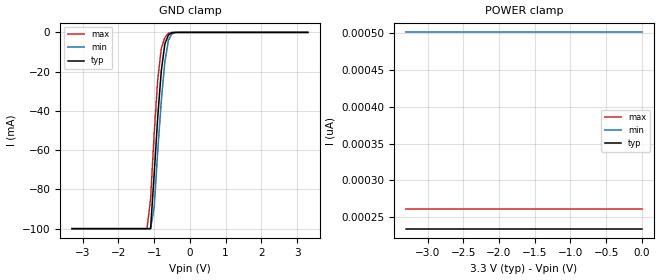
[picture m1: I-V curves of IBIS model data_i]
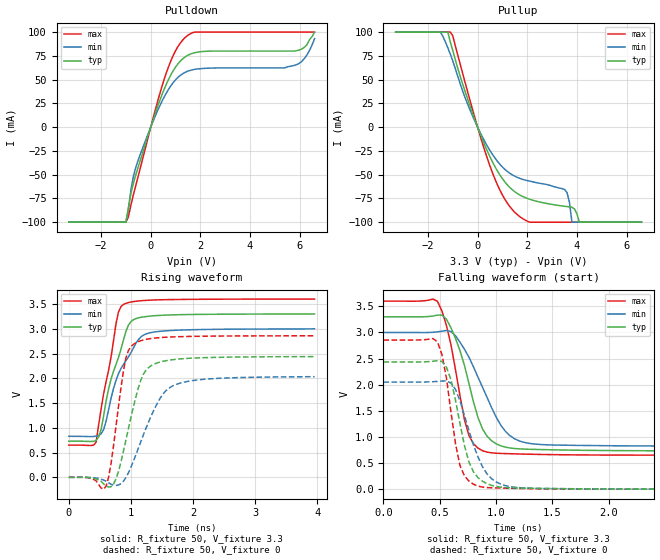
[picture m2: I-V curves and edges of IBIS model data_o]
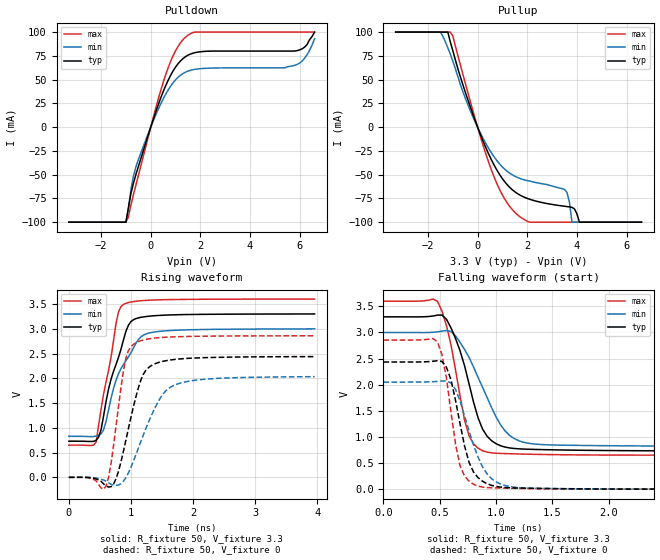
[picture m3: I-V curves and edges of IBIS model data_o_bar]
|   ON Semiconductor Corporation
|   IBIS Model of NL17SZ74DF
|   Single D type Flip-Flop
|   US8 (US) Package Type
[IBIS Ver]   3.2
[Comment Char]   |_char
[File name]   nl17sz74df_c300.ibs
[File Rev]   1.0
[Date]   06/15/04
[Source]
From lab measurements at ON Semiconductor
[Notes]
Created by Duane Mattheisen
Modeling Support Engineer
| This model represents the NL27WZ08DF where 3.0 <= Vcc =< 3.6
[Disclaimer]
ON Semiconductor Corporation hereby grants
the user of this IBIS model a license to use this IBIS
model under the following terms. This license in non-exclusive
and non-transferable. Before using this IBIS model. After reading
the terms and conditions of this license, the user either must accept
these terms, or the IBIS model should be returned to ON within 30 days.
   The user is hereby granted a license to use the
IBIS model. This shall not be construed as a right to sell, or otherwise
profit either by leasing or renting this software.
   The user may modify the IBIS model to suit his specific applications
but rights to derivative works and such modifications shall belong to
ON Semiconductor.
   This IBIS model is provided on an "as is" basis. ON Semiconductor
makes absolutely no warranty with respect to the information contained
herein. By use of this IBIS model, the user assumes full risk as to the
quality and suitability of the model to his particular use, and by using
this model assumes the entire risk. Under all circumstances the user shall
not hold ON Semiconductor liable in any way for the results obtained. ON
Semiconductor reserves the right to make to improve the model for reliability,
function, or design. ON Semiconductor does not convey any license under patent
rights or any other intellectual property rights, including those of third
parties.
ON Semiconductor is not obligated to provide maintenance or support
for the licensed IBIS model.
Cont ON at ATTN:LOGIC APPLICATIONS/IBIS MODEL.
5005 E. McDowell Road, Phoenix AZ 85008
[Copyright]
(c) 2002 ON Semiconductor Corp.
[Component]   NL17SZ74DF
Si_location Pin
Timing_location Pin
[Manufacturer]   ON Semiconductor Corp.
[Package]
|   typ   min   max
R_pkg   0.023   0.021   0.024
L_pkg   1.28nH   1.25nH   1.32nH
C_pkg   0.12pF   0.10pF   0.14pF
[Pin] signal_name   model_name   R_pin   L_pin   C_pin
1   CP   cntrl_i   24m   1.28n   0.11p
2   D   data_i   21m   1.26n   0.13p
3   Q_bar   data_o_bar   21m   1.25n   0.10p
4   GND   GND   24m   1.27n   0.12p
5   Q   data_o   24m   1.27n   0.14p
6   CLR   cntrl_i   21m   1.26n   0.13p
7   PR_bar   cntrl_i   21m   1.26n   0.10p
8   VCC   POWER   24m   1.32n   0.11p
| Models and submodels in the file (4): data_i (Input), cntrl_i (Input), data_o (Output), data_o_bar (Output)
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[Model]   data_i
Model_type Input
Vinh=2.31
Vinl=0.99
| variable   typ   min   max
C_comp   4.1pf   4.1pf   4.1pf
[Temperature Range] 25   85   -40
[Voltage Range]   3.3   3.00   3.6
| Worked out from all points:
|   GND clamp passes 1 mA (typ) near -0.57 V on its own axis
[GND Clamp]
-3.3V     -100mA     -100mA     -100mA
-1.2V     -100mA     -100mA     -100mA
-1.1V     -100mA     -100mA     -84.93mA
-1V       -72.43mA   -89.41mA   -51.83mA
-900mV    -43.25mA   -60.61mA   -24.15mA
-800mV    -19.56mA   -34.89mA   -8.202mA
-700mV    -5.809mA   -14.91mA   -2.618mA
-600mV    -1.337mA   -4.008mA   -423.3uA
-500mV    -147.5uA   -668uA     -11.99uA
-400mV    -5.049uA   -53.16uA   -112.1nA
3.3V      7pA        891.8pA    308.2pA
[POWER Clamp]
-3.3V     234.3pA    501pA      261.7pA
-3.2V     234.3pA    501pA      261.7pA
-3.1V     234.3pA    501pA      261.7pA
0V        234.3pA    501pA      261.7pA
[Model]   data_o
Model_type Output
Polarity Non-Inverting
Vref=0
Vmeas=1.65
Cref=50p
Rref=500
| variable   typ   min   max
C_comp   5.2pf   5.2pf   5.2pf
[Temperature Range] 25   85   -40
[Voltage Range]   3.3   3.0   3.6
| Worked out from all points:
|   slope of the pulldown table from 0 to 0.495 V, typ, clamps not added: 13.4 ohm
|   slope of the pullup table from 0 to 0.495 V, typ, clamps not added: 15.9 ohm
|   falling waveform, R_fixture 50, V_fixture 3.3: 20-80 % time 206ps typ, 284ps min, 158ps max; typ from 3.3 V to 0.732 V
|   falling waveform, R_fixture 50, V_fixture 0: 20-80 % time 151ps typ, 198ps min, 123ps max; typ from 2.44 V to 0 V
|   rising waveform, R_fixture 50, V_fixture 3.3: 20-80 % time 322ps typ, 398ps min, 247ps max; typ from 0.73 V to 3.3 V
|   rising waveform, R_fixture 50, V_fixture 0: 20-80 % time 284ps typ, 421ps min, 188ps max; typ from 0 V to 2.44 V
[Pullup]
-3.3V     99.99mA    99.99mA    99.99mA
-1.5V     99.99mA    99.99mA    99.99mA
-1.2V     99.99mA    83.48mA    99.99mA
-1.1V     89.6mA     76.82mA    99.99mA
-300mV    21.71mA    17.72mA    27.51mA
600mV     -36.68mA   -28.79mA   -48.1mA
1.7V      -71.4mA    -53.92mA   -94.2mA
3.5V      -83.23mA   -65.55mA   -99.99mA
3.7V      -83.9mA    -79.27mA   -99.99mA
3.8V      -84.35mA   -100mA     -99.99mA
4.1V      -100mA     -100mA     -99.99mA
6.6V      -100mA     -100mA     -99.99mA
[Pulldown]
-3.3V     -100mA     -100mA     -100mA
-1V       -100mA     -100mA     -100mA
-900mV    -84.8mA    -86.46mA   -94.46mA
-800mV    -70.01mA   -66.1mA    -82.18mA
-600mV    -50.06mA   -42.1mA    -61.16mA
100mV     8.01mA     6.458mA    9.967mA
800mV     54.47mA    43.09mA    69.09mA
1.1V      66.72mA    52.43mA    84.98mA
1.5V      75.69mA    58.96mA    96.72mA
5.4V      80.03mA    62.33mA    99.99mA
6.1V      82.41mA    69.59mA    99.99mA
6.6V      99.99mA    93.09mA    99.99mA
[Ramp]
dV/dt_r  1.46E+00/2.80E-10  1.22E+00/4.40E-10  1.71E+00/2.00E-10
dV/dt_f  1.54E+00/2.00E-10 1.31E+00/2.80E-10  1.77E+00/1.60E-10
[Falling Waveform]
R_fixture=50
C_fixture=0p
V_fixture=3.3
V_fixture_min=3.0
V_fixture_max=3.6
|Time   Typ   Min   Max
|SECONDS   VOLTS   VOLTS   VOLTS
0s        3.3V       3V         3.6V
480ps     3.333V     3.012V     3.597V
520ps     3.333V     3.026V     3.409V
600ps     3.088V     3.018V     2.763V
720ps     2.366V     2.677V     1.327V
760ps     2.019V     2.525V     1.024V
880ps     1.152V     1.952V     736.5mV
1.08ns    806mV      1.116V     681.4mV
1.28ns    764.9mV    881.8mV    670mV
3.96ns    731.6mV    822.2mV    650.8mV
[Falling Waveform]
R_fixture=50
C_fixture=0p
V_fixture=0
|Time   Typ   Min   Max
|SECONDS   VOLTS   VOLTS   VOLTS
0s        2.435V     2.05V      2.855V
480ps     2.46V      2.063V     2.82V
520ps     2.445V     2.071V     2.574V
600ps     2.095V     2.031V     1.471V
680ps     1.257V     1.692V     450.5mV
760ps     516mV      1.117V     153.5mV
840ps     220.3mV    615.1mV    58.45mV
960ps     72.88mV    200.6mV    26.28mV
1.2ns     21.59mV    30.4mV     13.28mV
3.96ns    0V         0V         0V
[Rising Waveform]
R_fixture=50
C_fixture=0p
V_fixture=3.3
V_fixture_min=3.0
V_fixture_max=3.6
|Time   Typ   Min   Max
|SECONDS   VOLTS   VOLTS   VOLTS
0s        730.3mV    828.5mV    650.6mV
440ps     746.3mV    832.8mV    712.8mV
560ps     1.237V     962.1mV    1.681V
640ps     1.78V      1.361V     2.158V
760ps     2.278V     1.958V     3.101V
880ps     2.772V     2.28V      3.491V
1ns       3.143V     2.516V     3.54V
1.16ns    3.231V     2.834V     3.566V
1.32ns    3.257V     2.923V     3.579V
3.96ns    3.3V       3V         3.6V
[Rising Waveform]
R_fixture=50
C_fixture=0p
V_fixture=0
|Time   Typ   Min   Max
|SECONDS   VOLTS   VOLTS   VOLTS
0s        0V         0V         0V
600ps     -174.3mV   -77.47mV   -178.4mV
680ps     -188.5mV   -139.1mV   276.9mV
760ps     -31.95mV   -162.8mV   1.03V
920ps     753.5mV    -4.039mV   2.409V
1.08ns    1.621V     453.9mV    2.716V
1.28ns    2.211V     1.103V     2.795V
1.52ns    2.344V     1.686V     2.826V
1.72ns    2.383V     1.872V     2.838V
3.96ns    2.438V     2.033V     2.858V
[Model]   data_o_bar
Model_type Output
Polarity Inverting
Vref=0
Vmeas=1.65
Cref=50p
Rref=500
| variable   typ   min   max
C_comp   5.2pf   5.2pf   5.2pf
[Temperature Range] 25   85   -40
[Voltage Range]   3.3   3.0   3.6
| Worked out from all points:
|   slope of the pulldown table from 0 to 0.495 V, typ, clamps not added: 13.4 ohm
|   slope of the pullup table from 0 to 0.495 V, typ, clamps not added: 15.9 ohm
|   falling waveform, R_fixture 50, V_fixture 3.3: 20-80 % time 206ps typ, 284ps min, 158ps max; typ from 3.3 V to 0.732 V
|   falling waveform, R_fixture 50, V_fixture 0: 20-80 % time 151ps typ, 198ps min, 123ps max; typ from 2.44 V to 0 V
|   rising waveform, R_fixture 50, V_fixture 3.3: 20-80 % time 322ps typ, 398ps min, 247ps max; typ from 0.73 V to 3.3 V
|   rising waveform, R_fixture 50, V_fixture 0: 20-80 % time 284ps typ, 421ps min, 188ps max; typ from 0 V to 2.44 V
[Pullup]
-3.3V     99.99mA    99.99mA    99.99mA
-1.5V     99.99mA    99.99mA    99.99mA
-1.2V     99.99mA    83.48mA    99.99mA
-1.1V     89.6mA     76.82mA    99.99mA
-300mV    21.71mA    17.72mA    27.51mA
600mV     -36.68mA   -28.79mA   -48.1mA
1.7V      -71.4mA    -53.92mA   -94.2mA
3.5V      -83.23mA   -65.55mA   -99.99mA
3.7V      -83.9mA    -79.27mA   -99.99mA
3.8V      -84.35mA   -100mA     -99.99mA
4.1V      -100mA     -100mA     -99.99mA
6.6V      -100mA     -100mA     -99.99mA
[Pulldown]
-3.3V     -100mA     -100mA     -100mA
-1V       -100mA     -100mA     -100mA
-900mV    -84.8mA    -86.46mA   -94.46mA
-800mV    -70.01mA   -66.1mA    -82.18mA
-600mV    -50.06mA   -42.1mA    -61.16mA
100mV     8.01mA     6.458mA    9.967mA
800mV     54.47mA    43.09mA    69.09mA
1.1V      66.72mA    52.43mA    84.98mA
1.5V      75.69mA    58.96mA    96.72mA
5.4V      80.03mA    62.33mA    99.99mA
6.1V      82.41mA    69.59mA    99.99mA
6.6V      99.99mA    93.09mA    99.99mA
[Ramp]
dV/dt_r  1.46E+00/2.80E-10  1.22E+00/4.40E-10  1.71E+00/2.00E-10
dV/dt_f  1.54E+00/2.00E-10 1.31E+00/2.80E-10  1.77E+00/1.60E-10
[Falling Waveform]
R_fixture=50
C_fixture=0p
V_fixture=3.3
V_fixture_min=3.0
V_fixture_max=3.6
|Time   Typ   Min   Max
|SECONDS   VOLTS   VOLTS   VOLTS
0s        3.3V       3V         3.6V
480ps     3.333V     3.012V     3.597V
520ps     3.333V     3.026V     3.409V
600ps     3.088V     3.018V     2.763V
720ps     2.366V     2.677V     1.327V
760ps     2.019V     2.525V     1.024V
880ps     1.152V     1.952V     736.5mV
1.08ns    806mV      1.116V     681.4mV
1.28ns    764.9mV    881.8mV    670mV
3.96ns    731.6mV    822.2mV    650.8mV
[Falling Waveform]
R_fixture=50
C_fixture=0p
V_fixture=0
|Time   Typ   Min   Max
|SECONDS   VOLTS   VOLTS   VOLTS
0s        2.435V     2.05V      2.855V
480ps     2.46V      2.063V     2.82V
520ps     2.445V     2.071V     2.574V
600ps     2.095V     2.031V     1.471V
680ps     1.257V     1.692V     450.5mV
760ps     516mV      1.117V     153.5mV
840ps     220.3mV    615.1mV    58.45mV
960ps     72.88mV    200.6mV    26.28mV
1.2ns     21.59mV    30.4mV     13.28mV
3.96ns    0V         0V         0V
[Rising Waveform]
R_fixture=50
C_fixture=0p
V_fixture=3.3
V_fixture_min=3.0
V_fixture_max=3.6
|Time   Typ   Min   Max
|SECONDS   VOLTS   VOLTS   VOLTS
0s        730.3mV    828.5mV    650.6mV
440ps     746.3mV    832.8mV    712.8mV
560ps     1.237V     962.1mV    1.681V
640ps     1.78V      1.361V     2.158V
760ps     2.278V     1.958V     3.101V
880ps     2.772V     2.28V      3.491V
1ns       3.143V     2.516V     3.54V
1.16ns    3.231V     2.834V     3.566V
1.32ns    3.257V     2.923V     3.579V
3.96ns    3.3V       3V         3.6V
[Rising Waveform]
R_fixture=50
C_fixture=0p
V_fixture=0
|Time   Typ   Min   Max
|SECONDS   VOLTS   VOLTS   VOLTS
0s        0V         0V         0V
600ps     -174.3mV   -77.47mV   -178.4mV
680ps     -188.5mV   -139.1mV   276.9mV
760ps     -31.95mV   -162.8mV   1.03V
920ps     753.5mV    -4.039mV   2.409V
1.08ns    1.621V     453.9mV    2.716V
1.28ns    2.211V     1.103V     2.795V
1.52ns    2.344V     1.686V     2.826V
1.72ns    2.383V     1.872V     2.838V
3.96ns    2.438V     2.033V     2.858V
